(* Logix 5000 AddOnInstructionDefinition export AMCI_MA_Reset_Driver_Fault; software revision 20.05 *)

TYPE AMCI_Motion_Axis_Output_Data :
STRUCT
   Control_Word_0 : INT;
   Control_Word_1 : INT;
   Position_or_Distance : DINT;
   Programmed_Speed : DINT;
   Acceleration : INT;
   Deceleration : INT;
   Output_Word_8 : INT;
   Output_Word_9 : INT;
END_STRUCT
END_TYPE

TYPE AMCI_Motion_Axis_Input_Data :
STRUCT
   Moving_CW : BOOL;
   Moving_CCW : BOOL;
   In_Hold_State : BOOL;
   Stopped : BOOL;
   At_Home : BOOL;
   Accelerating : BOOL;
   Decelerating : BOOL;
   Move_Complete : BOOL;
   Status_Word_0_Bit_8 : BOOL;
   Status_Word_0_Bit_9 : BOOL;
   Position_Invalid : BOOL;
   Input_Error : BOOL;
   Command_Error : BOOL;
   Configuration_Error : BOOL;
   Module_OK : BOOL;
   Mode_Flag : BOOL;
   IN1_Active : BOOL;
   IN2_Active : BOOL;
   IN3_Active : BOOL;
   IN4_Active : BOOL;
   Status_Word_1_Bit_4 : BOOL;
   Status_Word_1_Bit_5 : BOOL;
   Connection_Was_Lost : BOOL;
   Driver_Fault : BOOL;
   Status_Word_1_Bit_8 : BOOL;
   Invalid_Jog_Change : BOOL;
   Status_Word_1_Bit_10 : BOOL;
   Heartbeat_Bit : BOOL;
   Status_Word_1_Bit_12 : BOOL;
   Status_Word_1_Bit_13 : BOOL;
   Stall_Detected : BOOL;
   Drive_Is_Enabled : BOOL;
   Motor_Position : DINT;
   Encoder_Position : DINT;
   Trapped_Encoder_Position : DINT;
   Input_Word_8 : INT;
   Input_Word_9 : INT;
END_STRUCT
END_TYPE

ADD_ON_INSTRUCTION AMCI_MA_Reset_Driver_Fault   (* revision 1.0, vendor AMCI, ExecuteEnableInFalse *)
// AMCI Reset Driver Faults.   Only for SDXXXXE2 and SMDXXE2 units.
// Help:
// MOTION AXIS RESET DRIVER FAULTS
// This AOI will only work with SMD34E2, SD4840E2, SD17060E2, and SMD31045E2 units.  This AOI WILL NOT WORK with SV160E2 and SV400E2 units.
// AXIS INPUT DATA:  Input data from AMCI motion device.   Uses the AMCI_Motion_Axis_Input_Data User Defined Data Type.
// AXIS OUTPUT DATA; Output data from the AOI to the AMCI motion device.   Uses the AMCI_Motion_Axis_Output_Data User Defined Data Type.
// EN (Enable) Set when rung is true, Reset when rung is false
// DN (Done) Set when command is sent to the motion device.  Reset when the rung is false.
// ER (Error)  The driver fault  failed to clear.  Reset when the rung is false.
VAR_IN_OUT
   Axis_Input_Data : AMCI_Motion_Axis_Input_Data; {required}
        [0].6   // set when decelerating
   Axis_Output_Data : AMCI_Motion_Axis_Output_Data; {required}
END_VAR
VAR_OUTPUT
   EN : BOOL; {visible}   // set when rung with AOI is true
   DN : BOOL; {access Read Only, visible}   // set when reset error command sent to motion axis
   ER : BOOL; {access Read Only, visible}   // set when reset error command did not clear the driver fault
END_VAR
VAR
   command_data_block : INT[10];
        [0]   // Command Bits MSW
        [1]   // Command Bits LSW
        [2]   // Upper Target Position
        [3]   // Lower Target Position
        [4]   // Upper Programmed Speed
        [5]   // Lower Programmed Speed
   Initialize_timer : TIMER := (PRE := 100); {access None}
END_VAR

ROUTINE EnableInFalse   (* ladder *)
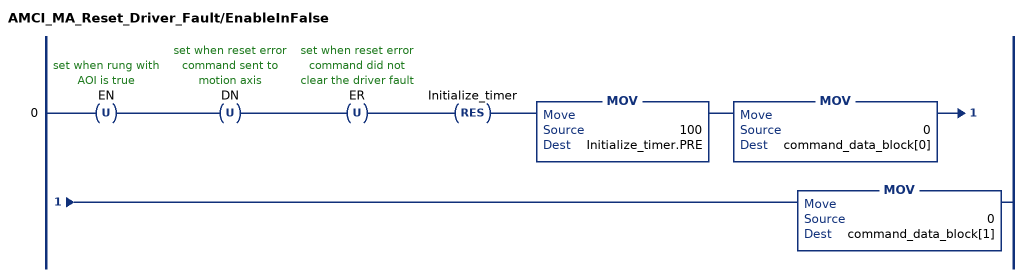
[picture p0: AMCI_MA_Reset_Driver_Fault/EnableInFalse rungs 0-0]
   0: OTU(EN)OTU(DN)OTU(ER)RES(Initialize_timer)MOV(100,Initialize_timer.PRE)MOV(0,command_data_block[0])MOV(0,command_data_block[1]);
END_ROUTINE

ROUTINE Logic   (* ladder *)
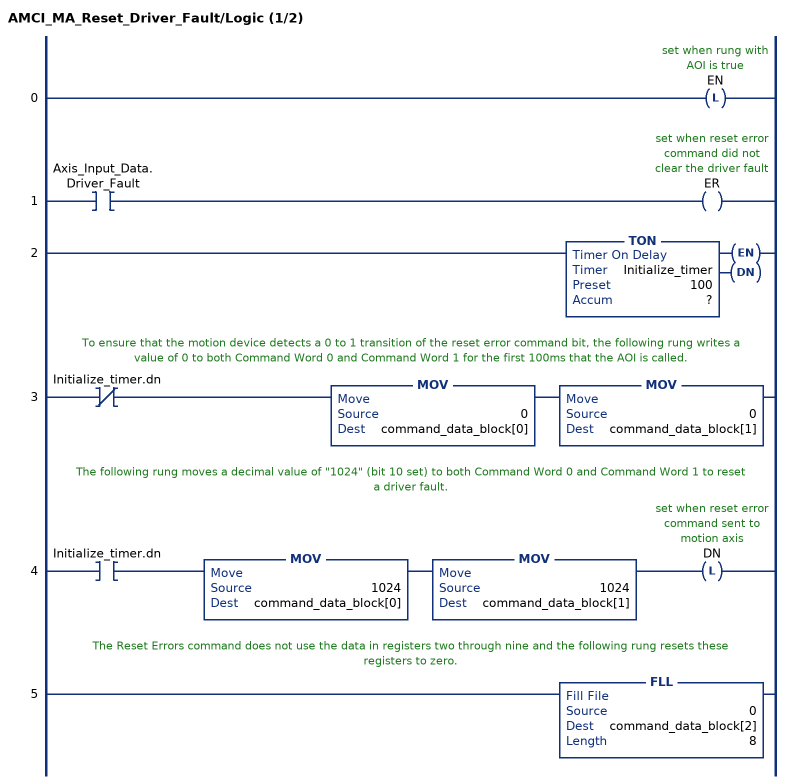
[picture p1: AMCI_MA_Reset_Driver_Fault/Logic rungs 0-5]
   0: OTL(EN);
   1: XIC(Axis_Input_Data.Driver_Fault)OTE(ER);
   2: TON(Initialize_timer,?,?);
   // To ensure that the motion device detects a 0 to 1 transition of the reset error command bit, the following rung writes a value of 0 to both Command Word 0 and Command Word 1 for the first 100ms that the AOI is called.
   3: XIO(Initialize_timer.dn)MOV(0,command_data_block[0])MOV(0,command_data_block[1]);
   // The following rung moves a decimal value of "1024" (bit 10 set) to both Command Word 0 and Command Word 1 to reset a driver fault.
   4: XIC(Initialize_timer.dn)MOV(1024,command_data_block[0])MOV(1024,command_data_block[1])OTL(DN);
   // The Reset Errors command does not use the data in registers two through nine and the following rung resets these registers to zero.
   5: FLL(0,command_data_block[2],8);
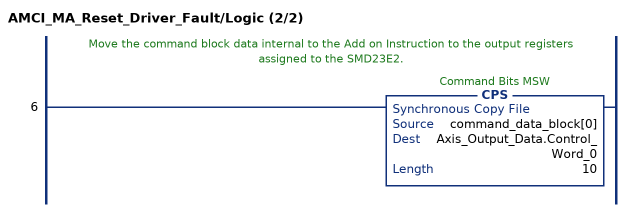
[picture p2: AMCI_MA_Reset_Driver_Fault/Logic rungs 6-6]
   // Move the command block data internal to the Add on Instruction to the output registers assigned to the SMD23E2.
   6: CPS(command_data_block[0],Axis_Output_Data.Control_Word_0,10);
END_ROUTINE
END_ADD_ON_INSTRUCTION
